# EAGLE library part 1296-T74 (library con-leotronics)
1.27mm SINGLE ROW FEMALE SOCKET Source: http://www.leotronics.co.uk/Conexcon/Data%20Sheets/sec.%20A/1296ing.pdf
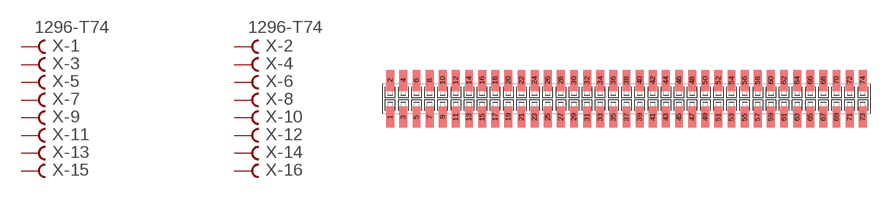
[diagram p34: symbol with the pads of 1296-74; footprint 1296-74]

Designator prefix X; gates -1=FVAL -2=FVAL -3=F -4=F -5=F -6=F -7=F -8=F -9=F -10=F -11=F -12=F -13=F -14=F -15=F -16=F -17=F -18=F -19=F -20=F -21=F -22=F -23=F -24=F -25=F -26=F -27=F -28=F -29=F -30=F -31=F -32=F -33=F -34=F -35=F -36=F -37=F -38=F -39=F -40=F -41=F -42=F -43=F -44=F -45=F -46=F -47=F -48=F -49=F -50=F -51=F -52=F -53=F -54=F -55=F -56=F -57=F -58=F -59=F -60=F -61=F -62=F -63=F -64=F -65=F -66=F -67=F -68=F -69=F -70=F -71=F -72=F -73=F -74=F

## 1296-T74 (OC_FARNELL: unknown; OC_NEWARK: unknown)  [1296-74]
1  -1:B  pas
2  -2:B  pas
3  -3:B  pas
4  -4:B  pas
5  -5:B  pas
6  -6:B  pas
7  -7:B  pas
8  -8:B  pas
9  -9:B  pas
10  -10:B  pas
11  -11:B  pas
12  -12:B  pas
13  -13:B  pas
14  -14:B  pas
15  -15:B  pas
16  -16:B  pas
17  -17:B  pas
18  -18:B  pas
19  -19:B  pas
20  -20:B  pas
21  -21:B  pas
22  -22:B  pas
23  -23:B  pas
24  -24:B  pas
25  -25:B  pas
26  -26:B  pas
27  -27:B  pas
28  -28:B  pas
29  -29:B  pas
30  -30:B  pas
31  -31:B  pas
32  -32:B  pas
33  -33:B  pas
34  -34:B  pas
35  -35:B  pas
36  -36:B  pas
37  -37:B  pas
38  -38:B  pas
39  -39:B  pas
40  -40:B  pas
41  -41:B  pas
42  -42:B  pas
43  -43:B  pas
44  -44:B  pas
45  -45:B  pas
46  -46:B  pas
47  -47:B  pas
48  -48:B  pas
49  -49:B  pas
50  -50:B  pas
51  -51:B  pas
52  -52:B  pas
53  -53:B  pas
54  -54:B  pas
55  -55:B  pas
56  -56:B  pas
57  -57:B  pas
58  -58:B  pas
59  -59:B  pas
60  -60:B  pas
61  -61:B  pas
62  -62:B  pas
63  -63:B  pas
64  -64:B  pas
65  -65:B  pas
66  -66:B  pas
67  -67:B  pas
68  -68:B  pas
69  -69:B  pas
70  -70:B  pas
71  -71:B  pas
72  -72:B  pas
73  -73:B  pas
74  -74:B  pas

## Footprint 1296-74 (pad centres in mm)
1.27mm SINGLE ROW FEMALE SOCKET Source: http://www.leotronics.co.uk/Conexcon/Data%20Sheets/sec.%20A/1296ing.pdf
smd 0.76 x 2.05: 1 -22.86,-1.78; 2 -22.86,1.78; 3 -21.59,-1.78; 4 -21.59,1.78; 5 -20.32,-1.78; 6 -20.32,1.78; 7 -19.05,-1.78; 8 -19.05,1.78; 9 -17.78,-1.78; 10 -17.78,1.78; 11 -16.51,-1.78; 12 -16.51,1.78; 13 -15.24,-1.78; 14 -15.24,1.78; 15 -13.97,-1.78; 16 -13.97,1.78; 17 -12.7,-1.78; 18 -12.7,1.78; 19 -11.43,-1.78; 20 -11.43,1.78; 21 -10.16,-1.78; 22 -10.16,1.78; 23 -8.89,-1.78; 24 -8.89,1.78; 25 -7.62,-1.78; 26 -7.62,1.78; 27 -6.35,-1.78; 28 -6.35,1.78; 29 -5.08,-1.78; 30 -5.08,1.78; 31 -3.81,-1.78; 32 -3.81,1.78; 33 -2.54,-1.78; 34 -2.54,1.78; 35 -1.27,-1.78; 36 -1.27,1.78; 37 0,-1.78; 38 0,1.78; 39 1.27,-1.78; 40 1.27,1.78; 41 2.54,-1.78; 42 2.54,1.78; 43 3.81,-1.78; 44 3.81,1.78; 45 5.08,-1.78; 46 5.08,1.78; 47 6.35,-1.78; 48 6.35,1.78; 49 7.62,-1.78; 50 7.62,1.78; 51 8.89,-1.78; 52 8.89,1.78; 53 10.16,-1.78; 54 10.16,1.78; 55 11.43,-1.78; 56 11.43,1.78; 57 12.7,-1.78; 58 12.7,1.78; 59 13.97,-1.78; 60 13.97,1.78; 61 15.24,-1.78; 62 15.24,1.78; 63 16.51,-1.78; 64 16.51,1.78; 65 17.78,-1.78; 66 17.78,1.78; 67 19.05,-1.78; 68 19.05,1.78; 69 20.32,-1.78; 70 20.32,1.78; 71 21.59,-1.78; 72 21.59,1.78; 73 22.86,-1.78; 74 22.86,1.78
